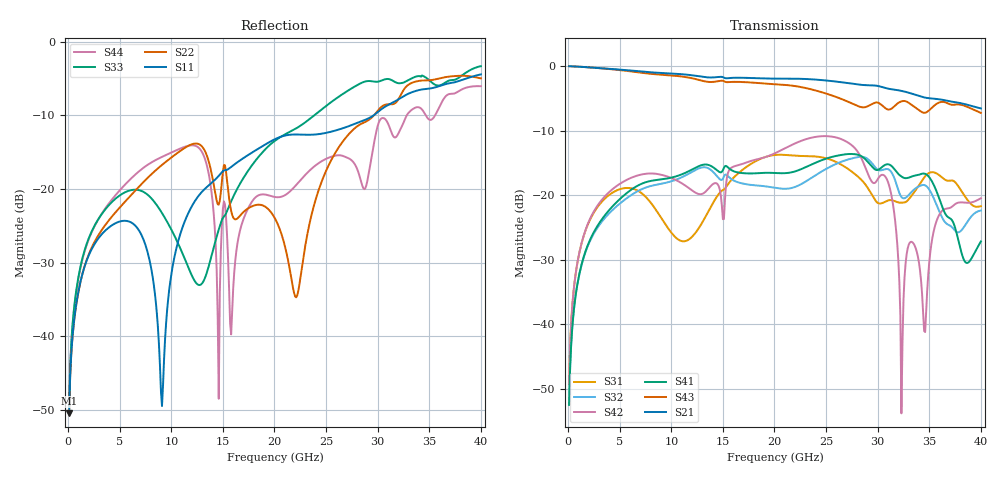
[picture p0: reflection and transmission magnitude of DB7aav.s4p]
! ADC12DJ2700AAV, ADC12DJ3200AAV, ADC08DJ3200AAV
! 144 pin AAV package
! Texas Instruments 4/21/2021
! Single-ended  S-parameters
! PORT#  PORT_NAME  NET_NAME
! PORT1:  DAxN.DIEBUMP DAxN
! PORT2:  DAxN.BGA  DAxN
! PORT3:  DAxP.DIEBUMP DAxP
! PORT4:  DAxP.BGA  DAxP
! Touchstone Ver. 1.0
! Number of ports is 4
# Hz	S	MA	R	50.000000
! SCATTERING PARAMETERS  :
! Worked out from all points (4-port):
!   400 points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, 100 MHz to 40 GHz, reference 50 ohm
!   strongest paths, dB at 100 MHz, 10.1 GHz, 20.1 GHz, 30.1 GHz, 40 GHz:
!     S21: 0.0, -1.2, -1.9, -3.1, -6.6
!     S43: 0.0, -1.5, -2.8, -5.7, -7.3
!     S41: -52.4, -17.2, -16.6, -16.0, -27.2
!     S42: -49.1, -17.4, -13.5, -17.3, -20.5
!     S32: -52.4, -17.8, -18.9, -16.1, -22.4
!     S31: -49.1, -26.0, -13.8, -21.3, -21.7
!   lowest |S11| = -50.5 dB at 100 MHz (marker M1), VSWR 1.01, Z = 50.1 + j0.263 ohm
!   |S11| at or under -10 dB: start of sweep to 29.59 GHz
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1e8  0.003001 61.0  0.9983 -1.3  0.003494 85.7  0.002388 -95.0
     0.9983 -1.3  0.002991 60.8  0.002388 -95.0  0.003492 86.2
     0.003494 85.7  0.002388 -95.0  0.003341 66.8  0.9985 -1.2
     0.002388 -95.0  0.003492 86.2  0.9985 -1.2  0.003324 67.0
7.2e9  0.04728 -59.0  0.9067 -80.2  0.1026 -44.9  0.1235 151.5
       0.9067 -80.2  0.1097 -21.5  0.112 157.6  0.1453 6.6
       0.1026 -44.9  0.112 157.6  0.09646 -61.8  0.886 -77.4
       0.1235 151.5  0.1453 6.6  0.886 -77.4  0.1377 -4.3
1.33e10  0.101 3.0  0.8205 -143.7  0.0679 152.1  0.1731 65.6
         0.8205 -143.7  0.1789 -123.9  0.1646 73.7  0.1062 -170.4
         0.0679 152.1  0.1646 73.7  0.02527 136.9  0.7601 -137.4
         0.1731 65.6  0.1062 -170.4  0.7601 -137.4  0.1574 -124.4
1.46e10  0.1229 -8.2  0.8238 -156.0  0.1023 124.5  0.1526 45.6
         0.8238 -156.0  0.07834 -117.2  0.1355 52.9  0.1175 96.2
         0.1023 124.5  0.1355 52.9  0.05305 92.1  0.765 -147.6
         0.1526 45.6  0.1175 96.2  0.765 -147.6  0.00376 -62.7
2.76e10  0.2742 -94.9  0.7295 62.7  0.1501 -70.3  0.2086 -112.6
         0.7295 62.7  0.2524 -25.4  0.1938 -74.7  0.2397 -51.2
         0.1501 -70.3  0.1938 -74.7  0.4892 -60.8  0.5103 81.0
         0.2086 -112.6  0.2397 -51.2  0.5103 81.0  0.1535 -60.3
3.23e10  0.4187 -123.1  0.6428 9.1  0.08762 151.4  0.1398 177.1
         0.6428 9.1  0.4441 -53.5  0.097 -152.0  0.002052 -164.2
         0.08762 151.4  0.097 -152.0  0.5253 -104.8  0.5329 47.0
         0.1398 177.1  0.002052 -164.2  0.5329 47.0  0.2631 -42.0
4e10  0.6015 143.4  0.4703 -73.3  0.08232 57.2  0.04387 141.5
      0.4703 -73.3  0.5651 -119.2  0.07618 169.9  0.09478 25.0
      0.08232 57.2  0.07618 169.9  0.684 -156.2  0.4339 -40.7
      0.04387 141.5  0.09478 25.0  0.4339 -40.7  0.5 -92.9
